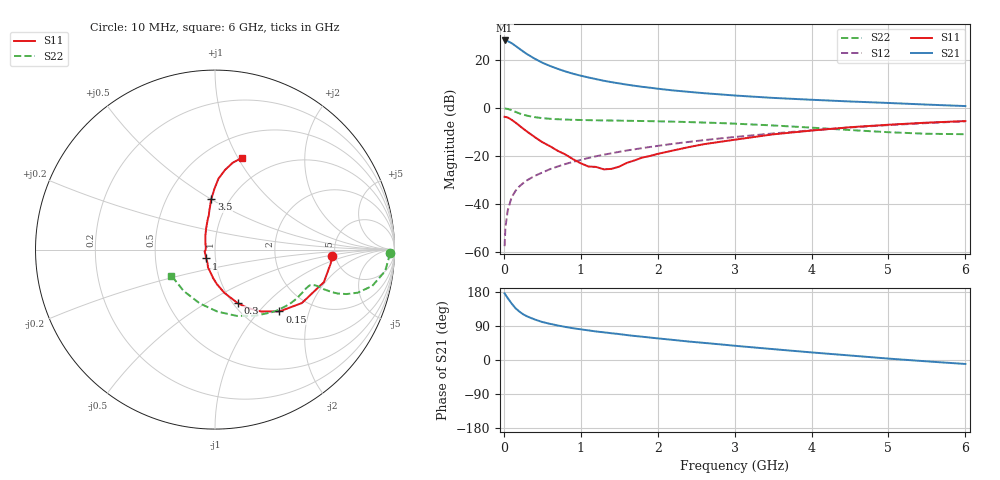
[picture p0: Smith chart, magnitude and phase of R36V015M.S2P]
! SIEMENS Small Signal Semiconductors
! BFR181
! Si NPN RF Bipolar Junction Transistor in SOT23
! VCE = 6 V  IC = 15 mA
! Common Emitter S-Parameters:  May  1996
# GHz  S  MA  R  50
!  f  S11  S21  S12  S22
! GHz  MAG  ANG  MAG  ANG  MAG  ANG  MAG  ANG
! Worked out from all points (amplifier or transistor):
!   36 points, 10 MHz to 6 GHz, reference 50 ohm
!   highest |S21| = 28.2 dB at 10 MHz (marker M1)
!   |S21| within 3 dB of that: start of sweep to 183.1 MHz
!   unconditionally stable (mu >= 1): 686.7 MHz to 2.604 GHz
!   at 250 MHz: K = 0.70, MSG = 27.5 dB, |S12| = -31.4 dB
!   at 1.4 GHz: K = 1.06, MAG = 13.4 dB, |S12| = -18.9 dB
!   at 6 GHz: K = 0.86, MSG = 3.2 dB, |S12| = -5.6 dB
!   S11 on the Smith chart (normalised r, x): 10 MHz: 4.69, -0.60; 150 MHz: 1.42, -1.30; 300 MHz: 1.05, -0.70; 1 GHz: 0.90, -0.09; 3.5 GHz: 0.82, +0.50; 6 GHz: 0.73, +1.04
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0.01  0.6536 -3.2  25.7 175.8  0.0013 93.3  0.9772 -1.2
0.02  0.6498 -6.7  25.34 172.7  0.0031 86.5  0.9691 -2.9
0.05  0.6333 -16.6  24.85 163.5  0.0072 80.4  0.9556 -7.2
0.1  0.5683 -31.6  22.63 149.4  0.0135 77.3  0.8994 -13.0
0.15  0.4977 -43.8  19.87 137.0  0.0184 72.1  0.8308 -16.8
0.2  0.43 -53.3  17.39 128.1  0.0229 71.2  0.7728 -18.7
0.25  0.3712 -61.0  15.19 120.8  0.0268 70.0  0.7257 -19.7
0.3  0.3229 -67.1  13.37 115.3  0.0308 70.8  0.6909 -20.0
0.4  0.2477 -77.6  10.73 107.1  0.038 71.0  0.6432 -20.0
0.5  0.1933 -86.8  8.819 100.2  0.0449 71.9  0.613 -19.6
0.6  0.1591 -93.8  7.544 95.5  0.0527 72.3  0.5947 -19.6
0.7  0.1275 -101.7  6.569 91.1  0.0599 72.9  0.5815 -19.9
0.8  0.1069 -111.5  5.793 87.3  0.0676 72.4  0.5732 -20.1
1  0.0699 -135.2  4.72 80.9  0.0823 72.4  0.5612 -21.1
1.1  0.06 -150.8  4.336 78.2  0.0903 72.2  0.5567 -22.0
1.3  0.0522 -178.2  3.701 73.0  0.1057 71.3  0.5495 -23.7
1.6  0.0715 138.4  3.067 65.7  0.1296 69.9  0.5403 -27.0
2.2  0.1294 112.3  2.326 53.0  0.1786 66.3  0.5181 -34.9
3.5  0.2811 94.3  1.624 28.7  0.2936 55.2  0.4315 -58.6
4.5  0.3961 87.2  1.367 11.9  0.3908 44.2  0.3458 -87.7
5.5  0.4937 78.5  1.176 -3.6  0.4838 31.3  0.2893 -127.1
6  0.5327 73.7  1.096 -10.5  0.5269 24.3  0.2832 -149.2
